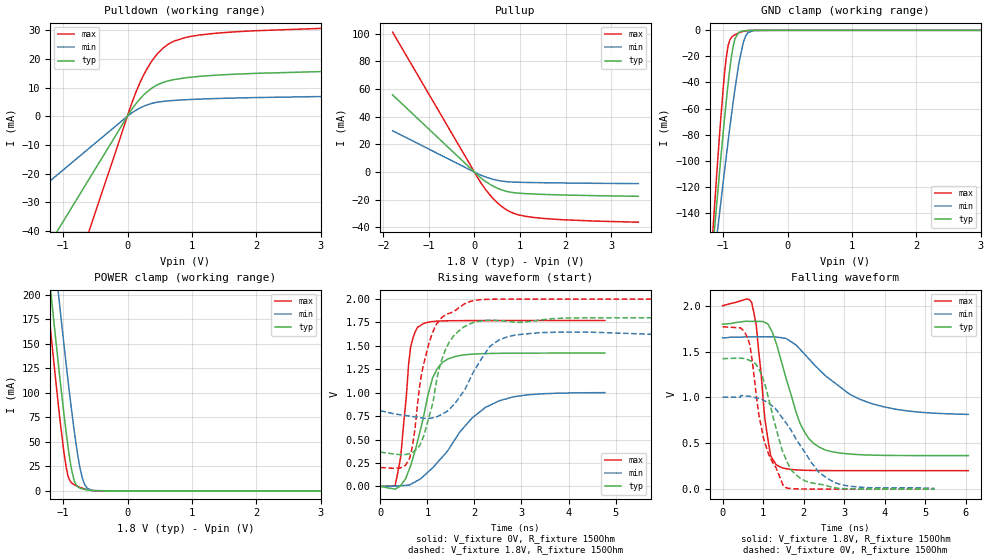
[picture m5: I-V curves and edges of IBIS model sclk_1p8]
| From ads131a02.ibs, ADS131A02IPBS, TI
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|   sclk_1p8 Model
[Model]   sclk_1p8
Model_type   I/O
Polarity   Non-Inverting
Enable   Active-Low
Vinl = 0.36
Vinh = 1.44
Vmeas = 0.9
Vref = 0
Cref = 2pF
Rref = 150
|   typ   min   max
|   (nom PVT)   (fast PVT)   (slow PVT)
C_comp   1.625e-12   1.609e-12   1.674e-12
| Where nom  PVT is Nominal Process, 1.8V, 27C
|   Fast PVT is Strong Process,  2V, -40C
|   Slow PVT is Weak Process,   1.65V, 125C
[Voltage Range]   1.8   1.65   2
|Junction Temperature
[Temperature Range]   27   125   -40
[Pullup Reference]   1.8   1.65   2
[Pulldown Reference]   0   0   0
[Power Clamp Reference]   1.8   1.65   2
[GND Clamp Reference]   0   0   0
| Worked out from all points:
|   slope of the pulldown table from 0 to 0.27 V, typ, clamps not added: 34.9 ohm
|   slope of the pullup table from 0 to 0.27 V, typ, clamps not added: 37.2 ohm
|   GND clamp passes 1 mA (typ) near -0.73 V on its own axis
|   POWER clamp passes 1 mA (typ) near -0.63 V on its own axis
|   falling waveform, V_fixture 1.8V, R_fixture 150Ohm: 20-80 % time 612ps typ, 1.38ns min, 251ps max; typ from 1.8 V to 0.366 V
|   rising waveform, V_fixture 0V, R_fixture 150Ohm: 20-80 % time 418ps typ, 1.01ns min, 187ps max; typ from 0 V to 1.42 V
|   rising waveform, V_fixture 1.8V, R_fixture 150Ohm: 20-80 % time 451ps typ, 595ps min, 390ps max; typ from 0.366 V to 1.8 V
|   falling waveform, V_fixture 0V, R_fixture 150Ohm: 20-80 % time 562ps typ, 906ps min, 440ps max; typ from 1.42 V to 0 V
[Pulldown]
|   Voltage   I(typ)   I(min)   I(max)
-1.8V     -66.16mA   -33.77mA   -120.8mA
-180mV    -6.616mA   -3.377mA   -12.08mA
62.85mV   2.259mA    1.079mA    4.339mA
142.2mV   4.681mA    2.22mA     9.014mA
252mV     7.429mA    3.471mA    14.42mA
358.2mV   9.465mA    4.336mA    18.57mA
437.4mV   10.61mA    4.774mA    21.04mA
554mV     11.79mA    5.166mA    23.79mA
638mV     12.35mA    5.347mA    25.18mA
898.2mV   13.38mA    5.735mA    27.44mA
1.368V    14.3mA     6.153mA    28.93mA
3.6V      15.93mA    7.06mA     31.11mA
[GND Clamp]
|   Voltage   I(typ)   I(min)   I(max)
-1.8V     -554.1mA   -474.7mA   -657.7mA
-1.148V   -160.7mA   -180.1mA   -145.4mA
-1.106V   -136.7mA   -161.9mA   -114.9mA
-1.055V   -108.2mA   -139.9mA   -79.28mA
-994mV    -75.58mA   -114.3mA   -41.37mA
-952.2mV  -54.57mA   -97.05mA   -21.15mA
-902mV    -31.92mA   -76.95mA   -8.255mA
-844.2mV  -12.3mA    -54.95mA   -4.252mA
-750.6mV  -1.393mA   -23.99mA   -1.807mA
-651.6mV  -214.4uA   -4.487mA   -445.2uA
-522.9mV  -14.93uA   -149.5uA   -26.28uA
3.6V      0A         0A         0A
[Pullup]
|   Voltage   I(typ)   I(min)   I(max)
-1.8V     55.83mA    29.89mA    101.2mA
59.4mV    -1.87mA    -984.1uA   -3.459mA
201.6mV   -5.723mA   -2.992mA   -10.64mA
360mV     -9.208mA   -4.757mA   -17.32mA
585.9mV   -12.72mA   -6.412mA   -24.51mA
731.1mV   -14.11mA   -6.966mA   -27.73mA
898.2mV   -14.98mA   -7.254mA   -30.19mA
1.33V     -15.86mA   -7.562mA   -32.85mA
1.98V     -16.55mA   -7.853mA   -34.46mA
3.6V      -17.47mA   -8.295mA   -36.17mA
[POWER Clamp]
|   Voltage   I(typ)   I(min)   I(max)
-1.8V     611.3mA    673.1mA    583.4mA
-1.411V   346.4mA    415.3mA    309.4mA
-1.208V   213.2mA    284.8mA    172.3mA
-1.168V   187.7mA    259.7mA    146.3mA
-1.069V   126mA      198.2mA    84.14mA
-989.9mV  79.46mA    150.4mA    40.13mA
-928.8mV  47.09mA    115mA      16.48mA
-838mV    12.59mA    66.16mA    6.746mA
-752.4mV  3.285mA    28.24mA    4.044mA
-668.1mV  1.506mA    6.791mA    2.06mA
-521.2mV  219.2uA    354.5uA    240.9uA
3.6V      0A         0A         0A
[Ramp]
R_load = 150
|   typ   min   max
dV/dt_r   0.854064/4.30048e-10   0.60067/9.81883e-10   1.06261/2.09145e-10
dV/dt_f   0.860453/6.25381e-10   0.503169/1.37569e-09   1.079/2.61171e-10
[Falling Waveform]
V_fixture = 1.8V
V_fixture_min = 1.65V
V_fixture_max = 2V
R_fixture = 150Ohm
|   Time   V(typ)   V(min)   V(max)
0s        1.8V       1.65V      2V
714.2ps   1.829V     1.661V     2.042V
835.1ps   1.829V     1.662V     1.776V
1.097ns   1.808V     1.662V     612.3mV
1.192ns   1.743V     1.662V     361.2mV
1.321ns   1.596V     1.66V      269mV
1.915ns   715.6mV    1.526V     208.2mV
2.396ns   456.4mV    1.3V       203.1mV
3.674ns   371.6mV    933.9mV    201.9mV
6.07ns    366.1mV    815.5mV    201.8mV
[Rising Waveform]
V_fixture = 0V
V_fixture_min = 0V
V_fixture_max = 0V
R_fixture = 150Ohm
|   Time   V(typ)   V(min)   V(max)
0s        1.048nV    65.85nV    185.3pV
314.2ps   -29.52mV   3.114mV    7.652mV
435.1ps   10.08mV    7.188mV    319mV
645.1ps   221.1mV    21.39mV    1.49V
791.8ps   480.6mV    62.55mV    1.699V
1.115ns   1.163V     199.3mV    1.76V
1.452ns   1.364V     395.6mV    1.768V
1.954ns   1.412V     731.6mV    1.77V
2.534ns   1.421V     915.1mV    1.771V
4.77ns    1.423V     1.001V     1.771V
[Rising Waveform]
V_fixture = 1.8V
V_fixture_min = 1.65V
V_fixture_max = 2V
R_fixture = 150Ohm
|   Time   V(typ)   V(min)   V(max)
0s        365.9mV    807.4mV    201.7mV
629.5ps   351.9mV    749.3mV    309.6mV
736.7ps   382.1mV    741.5mV    611mV
837.6ps   435mV      734mV      1.072V
1.091ns   841.3mV    729.2mV    1.614V
1.378ns   1.453V     789.8mV    1.828V
1.945ns   1.743V     1.188V     1.98V
2.516ns   1.77V      1.561V     1.999V
3.289ns   1.769V     1.637V     2V
13.27ns   1.8V       1.65V      2V
[Falling Waveform]
|Gnd
V_fixture = 0V
V_fixture_min = 0V
V_fixture_max = 0V
R_fixture = 150Ohm
|   Time   V(typ)   V(min)   V(max)
0s        1.423V     1.003V     1.771V
620.9ps   1.413V     1.014V     1.648V
678.7ps   1.402V     1.011V     1.564V
896.5ps   1.311V     988.8mV    811mV
1.014ns   1.186V     968.1mV    550.4mV
1.555ns   338.4mV    730.1mV    19.78mV
1.917ns   121.2mV    478mV      2.608mV
2.372ns   55.55mV    186.8mV    699.5uV
2.789ns   14.02mV    68.75mV    290.2uV
5.241ns   92.94uV    7.99mV     8.231uV
